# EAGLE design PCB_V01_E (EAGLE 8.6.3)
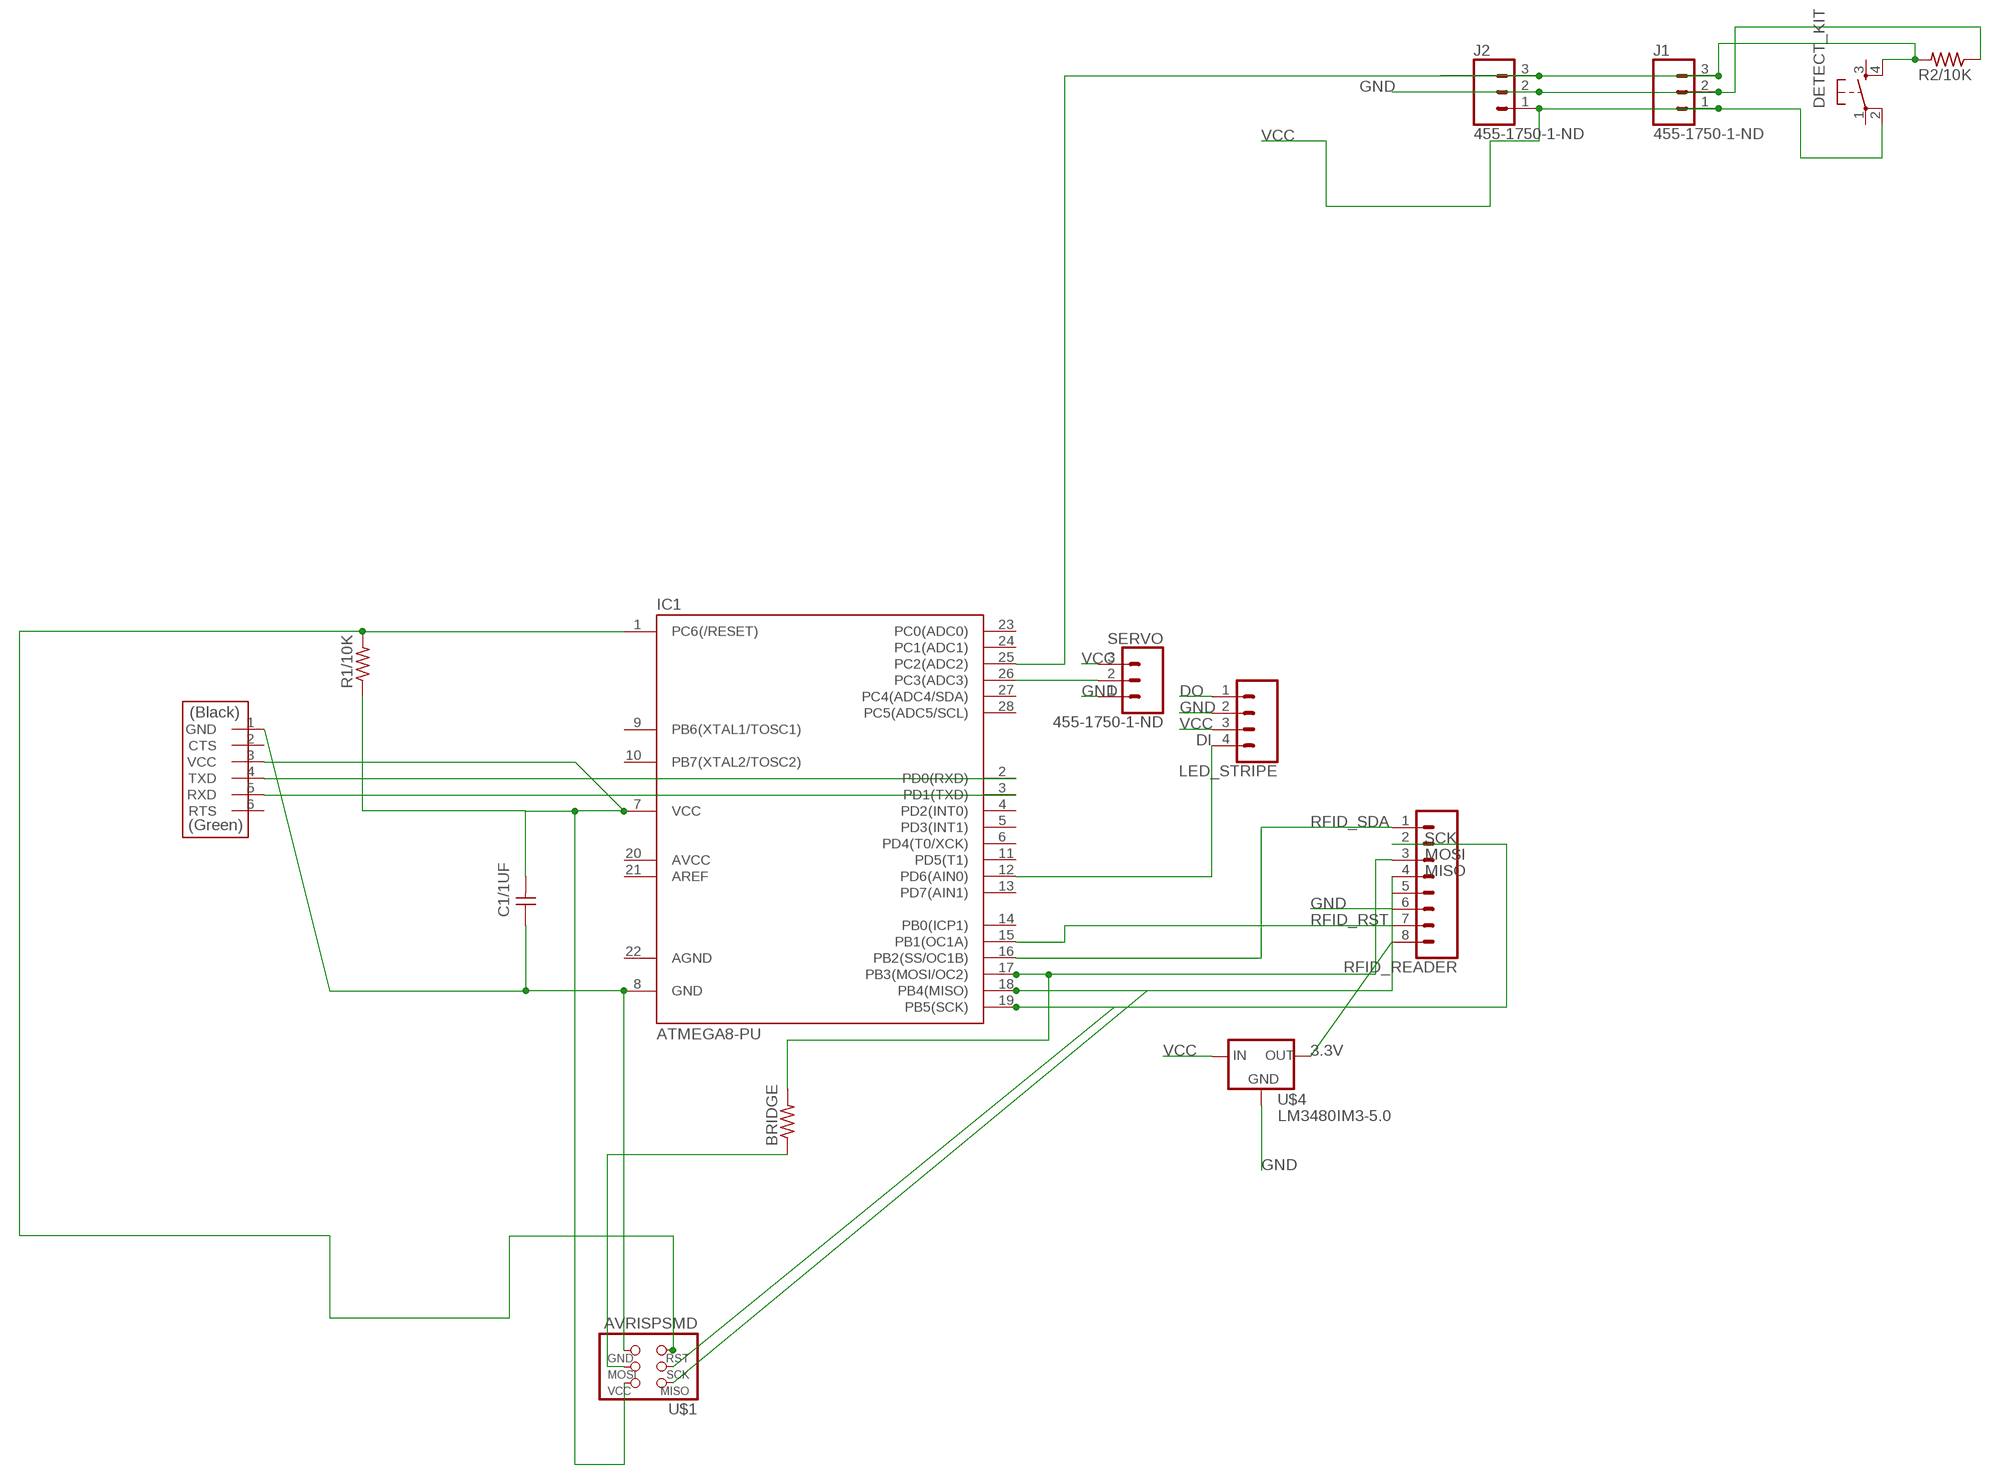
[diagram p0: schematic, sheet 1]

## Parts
BRIDGE  RES-US1206FAB  [R1206FAB]
C1/1UF  CAP-UNPOLARIZEDFAB  [C1206FAB]
DETECT_KIT  6MM_SWITCH6MM_SWITCH  [6MM_SWITCH]
IC1  ATMEGA8-PU  [DIL28-3]
J1  455-1750-1-ND  CONN_03  [1X03]
J2  455-1750-1-ND  CONN_03  [1X03]
LED_STRIPE  CONN_04  [1X04]
R1/10K  RES-US1206FAB  [R1206FAB]
R2/10K  RES-US1206FAB  [R1206FAB]
RFID_READER  CONN_08"  [1X08]
SERVO  455-1750-1-ND  CONN_03  [1X03]
U$1  AVRISPSMD  [2X03SMD]
U$2  FTDI-SMD-HEADER  [1X06SMD]
U$4  LM3480IM3-5.0  [SOT23]

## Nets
3.3V: RFID_READER.8 U$4.1(OUT)
DI: IC1.12(PD6(AIN0)) LED_STRIPE.4
DO: LED_STRIPE.1
GND: C1/1UF.1 IC1.8(GND) J1.2 J2.2 LED_STRIPE.2 R2/10K.1 RFID_READER.6 SERVO.1 U$1.6(GND) U$2.1(GND) U$4.3(GND)
MISO: IC1.18(PB4(MISO)) RFID_READER.4 U$1.1(MISO)
MOSI: BRIDGE.2 IC1.17(PB3(MOSI/OC2)) RFID_READER.3
N$1: BRIDGE.1 U$1.4(MOSI)
N$4: IC1.26(PC3(ADC3)) SERVO.2
N$8: IC1.3(PD1(TXD)) U$2.5(RXD)
N$9: IC1.2(PD0(RXD)) U$2.4(TXD)
N$10: DETECT_KIT.4(S1) IC1.25(PC2(ADC2)) J1.3 J2.3 R2/10K.2
N$14: IC1.1(PC6(/RESET)) R1/10K.2 U$1.5(RST)
RFID_RST: IC1.15(PB1(OC1A)) RFID_READER.7
RFID_SDA: IC1.16(PB2(SS/OC1B)) RFID_READER.1
SCK: IC1.19(PB5(SCK)) RFID_READER.2 U$1.3(SCK)
VCC: C1/1UF.2 DETECT_KIT.2(P1) IC1.7(VCC) J1.1 J2.1 LED_STRIPE.3 R1/10K.1 SERVO.3 U$1.2(VCC) U$2.3(VCC) U$4.2(IN)
Unconnected: DETECT_KIT.1(P) DETECT_KIT.3(S) IC1.4(PD2(INT0)) IC1.5(PD3(INT1)) IC1.6(PD4(T0/XCK)) IC1.9(PB6(XTAL1/TOSC1)) IC1.10(PB7(XTAL2/TOSC2)) IC1.11(PD5(T1)) IC1.13(PD7(AIN1)) IC1.14(PB0(ICP1)) IC1.20(AVCC) IC1.21(AREF) IC1.23(PC0(ADC0)) IC1.24(PC1(ADC1)) IC1.27(PC4(ADC4/SDA)) IC1.28(PC5(ADC5/SCL)) RFID_READER.5 U$2.2(CTS) U$2.6(RTS)

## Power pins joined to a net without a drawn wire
AGND: IC1.22(AGND)

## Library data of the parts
BRIDGE R1/10K R2/10K = fab:RES-US: Resistor (US Symbol)
C1/1UF = fab:CAP-UNPOLARIZED
DETECT_KIT = fab:6MM_SWITCH: OMRON SWITCH
IC1 = atmega8:ATMEGA8-PU
J1 J2 SERVO = SparkFun-Connectors:CONN_03: Multi connection point. Often used as Generic Header-pin footprint for 0.1 inch spaced/style header connections On any of the 0.1 inch spaced packages, you can populate with these: Break Away Headers - Straight (PRT-00116) Break Away Male Headers - Right Angle (PRT-00553) Female Headers (PRT-00115)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; PROD_ID: XXX-00000
LED_STRIPE = SparkFun-Connectors:CONN_04: Multi connection point. Often used as Generic Header-pin footprint for 0.1 inch spaced/style header connections On any of the 0.1 inch spaced packages, you can populate with these: Break Away Headers - Straight (PRT-00116) Break Away Male Headers - Right Angle (PRT-00553) Female Headers (PRT-00115)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; PROD_ID: CONN-09696
RFID_READER = SparkFun-Connectors:CONN_08: Multi connection point. Often used as Generic Header-pin footprint for 0.1 inch spaced/style header connections On any of the 0.1 inch spaced packages, you can populate with these: Break Away Headers - Straight (PRT-00116) Break Away Male Headers - Right Angle (PRT-00553) Female Headers (PRT-00115)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; PROD_ID: CONN-08438
U$1 = fab:AVRISP
U$2 = fab:FTDI-SMD-HEADER
U$4 = national_gaui:LM3480

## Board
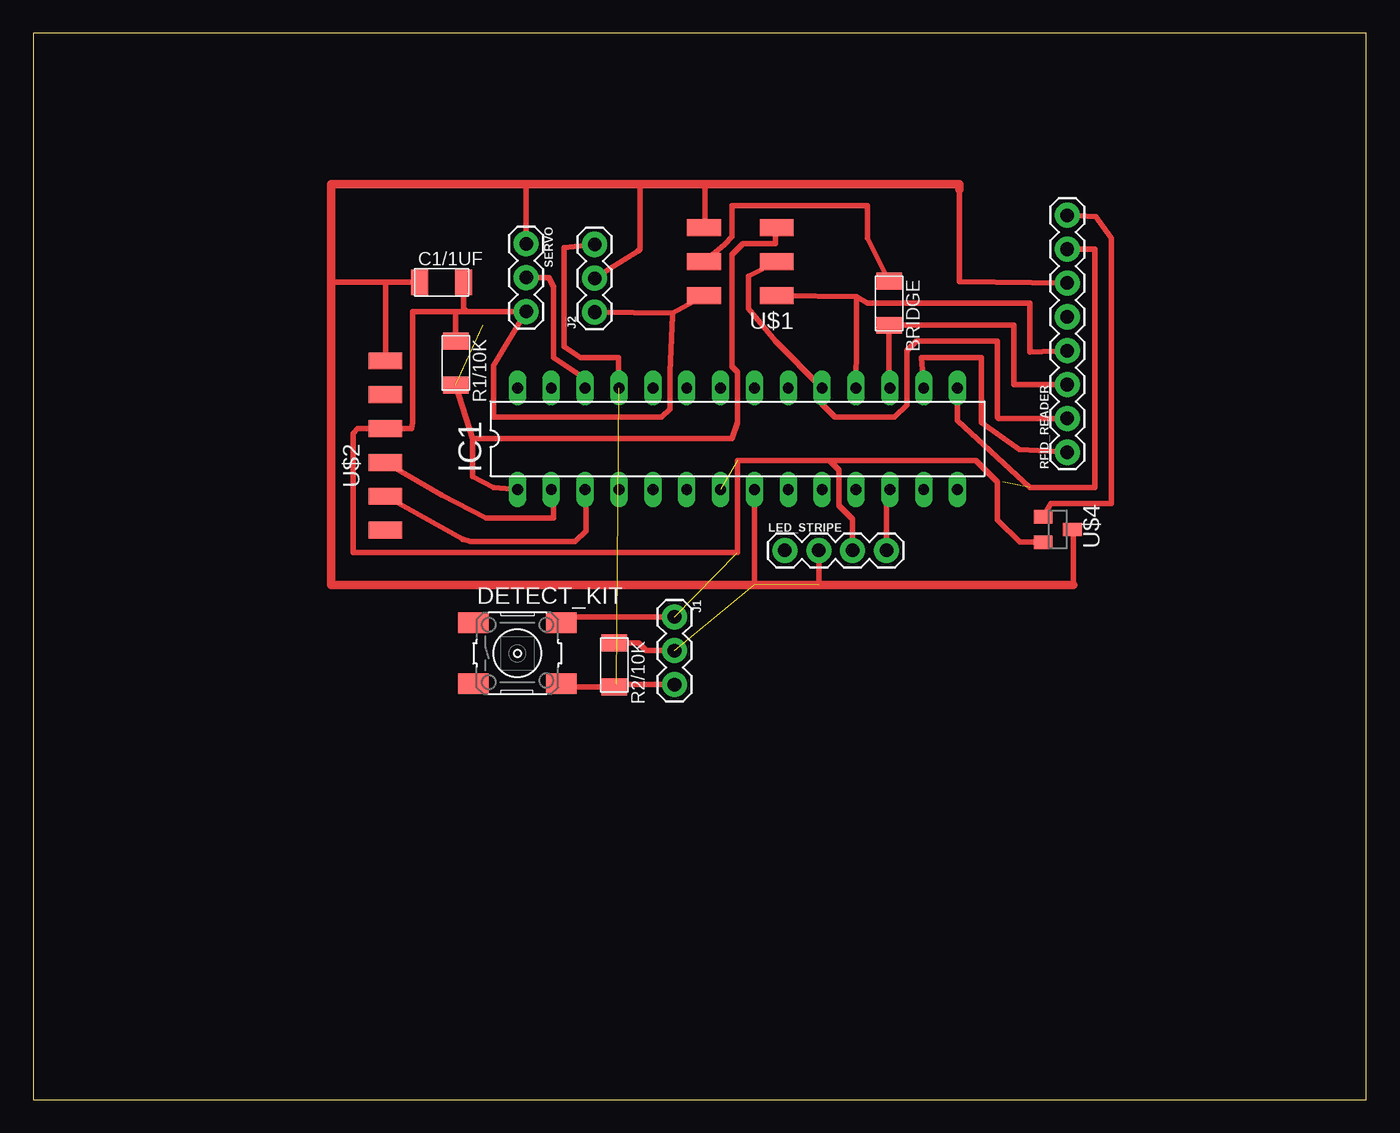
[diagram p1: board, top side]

Size 100 x 80 mm. Coordinates in mm from the lower left corner, seen from the top.
Outline: 0,0 100,0 100,80 0,80 0,0
Copper layers (1*16): Top 0.035mm / dielectric 1.5mm / Bottom 0.035mm
Design rules "default *": minimum track width 6mil, minimum drill 0.35mm, track to track 16mil, track to pad 16mil, pad to pad 16mil, via to via 16mil, smd to smd 16mil, copper to edge 40mil, drill to drill 6mil, minimum pad ring 10mil, minimum via ring 8mil, stop-mask expansion 4mil, vias tented up to drill 0mil, thermal gap 10mil

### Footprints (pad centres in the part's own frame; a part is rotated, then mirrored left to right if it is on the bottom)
R1206FAB = smd 1.27 x 1.905: 1 -1.651,0; 2 1.651,0
C1206FAB = smd 1.27 x 1.905: 1 -1.651,0; 2 1.651,0
6MM_SWITCH = smd 2.286 x 1.524: 1 -3.302,2.286; 2 3.302,2.286; 3 -3.302,-2.286; 4 3.302,-2.286
DIL28-3 = drill 0.813 long: 1 -16.51,-3.81; 2 -13.97,-3.81; 3 -11.43,-3.81; 4 -8.89,-3.81; 5 -6.35,-3.81; 6 -3.81,-3.81; 7 -1.27,-3.81; 8 1.27,-3.81; 9 3.81,-3.81; 10 6.35,-3.81; 11 8.89,-3.81; 12 11.43,-3.81; 13 13.97,-3.81; 14 16.51,-3.81; 15 16.51,3.81; 16 13.97,3.81; 17 11.43,3.81; 18 8.89,3.81; 19 6.35,3.81; 20 3.81,3.81; 21 1.27,3.81; 22 -1.27,3.81; 23 -3.81,3.81; 24 -6.35,3.81; 25 -8.89,3.81; 26 -11.43,3.81; 27 -13.97,3.81; 28 -16.51,3.81
1X03 = drill 1.016 pad 1.88: 1 0,0; 2 2.54,0; 3 5.08,0
1X04 = drill 1.016 pad 1.88: 1 0,0; 2 2.54,0; 3 5.08,0; 4 7.62,0
1X08 = drill 1.016 pad 1.88: 1 0,0; 2 2.54,0; 3 5.08,0; 4 7.62,0; 5 10.16,0; 6 12.7,0; 7 15.24,0; 8 17.78,0
2X03SMD = smd 2.54 x 1.27: 1 -2.54,2.54; 2 2.92,2.54; 3 -2.54,0; 4 2.92,0; 5 -2.54,-2.54; 6 2.92,-2.54
1X06SMD = smd 2.54 x 1.27: 1 0,6.35; 2 0,3.81; 3 0,1.27; 4 0,-1.27; 5 0,-3.81; 6 0,-6.35
SOT23 = smd 1 x 1.4: 1 -0.95,-1.1; 2 0.95,-1.1; 3 0,1.1

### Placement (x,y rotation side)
BRIDGE  64.21,59.74 270 top
C1/1UF  30.63,61.32 0 top
DETECT_KIT  36.32,33.48 0 top
IC1  52.83,49.58 0 top
J1  48.11,36.22 270 top
J2  42.11,59.08 90 top
LED_STRIPE  56.39,41.2 0 top
R1/10K  31.7,55.27 270 top
R2/10K  43.59,32.61 270 top
RFID_READER  77.57,48.56 90 top
SERVO  36.98,64.21 270 top
U$1  53.24,62.86 180 top
U$2  26.42,49.07 0 top
U$4  76.86,42.77 270 top

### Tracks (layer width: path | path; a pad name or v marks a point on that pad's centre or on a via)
3.3V
  Top 0.406: 75.95,43.91 U$4.1 76.33,44.7 80.87,44.7 80.87,64.62 79.7,66.24 RFID_READER.8
DI
  Top 0.406: LED_STRIPE.4 64.01,45.52 IC1.12
GND  (2 unrouted)
  Top 0.406: U$1.6 50.39,65.48 50.39,68.68 | SERVO.1 36.98,68.68 | J2.2 45.36,63.65 45.52,63.8 45.52,68.68 | RFID_READER.6 69.49,61.37 69.49,68.68 | 54.1,45.21 IC1.8 54.1,38.66 54.05,38.61 | LED_STRIPE.2 58.93,38.61 | J1.2 45.97,33.68 45.39,34.27 R2/10K.1 | U$4.3 78.03,42.77 78.03,38.61 | 22.35,61.37 22.35,61.32 26.42,61.32 | 26.42,61.32 C1/1UF.1 | U$2.1 26.42,61.32
  Top 0.635: 69.49,68.28 69.49,68.68 50.39,68.68 45.52,68.68 36.98,68.68 22.35,68.68 22.35,61.37 22.35,38.61 58.93,38.61 78.03,38.61
MISO
  Top 0.406: U$1.1 61.77,60.25 | 61.77,60.25 61.75,56.9 IC1.18 | RFID_READER.4 74.78,56.08 74.78,59.74 62.59,59.74 61.77,60.25
MOSI
  Top 0.406: IC1.17 64.35,53.39 64.21,53.52 BRIDGE.2 66.62,58.09 73.56,58.12 73.56,53.65 RFID_READER.3
N$1
  Top 0.406: U$1.4 51.84,64.16 52.43,64.74 52.43,67.06 62.59,67.06 62.59,64.64 BRIDGE.1
N$4
  Top 0.406: SERVO.2 38.71,61.67 39.01,60.96 39.01,55.68 41.4,54.1 IC1.26
N$8
  Top 0.406: U$2.5 32.21,42.04 | 32.21,42.04 32.26,42.01 | 32.21,42.04 32.79,41.86 40.64,41.86 41.45,42.67 41.45,45.72 IC1.3
N$9
  Top 0.406: U$2.4 30.63,45.36 33.98,43.64 39.01,43.64 39.01,45.62 IC1.2
N$10  (1 unrouted)
  Top 0.406: J2.3 39.83,63.91 39.83,56.49 41.05,55.68 43.89,55.68 43.94,53.59 IC1.25 | J1.3 43.76,31.14 R2/10K.2 39.85,30.96 DETECT_KIT.4
N$14  (1 unrouted)
  Top 0.406: R1/10K.2 32.94,49.58 | 32.94,49.58 32.94,46.76 34.54,45.92 IC1.1 | U$1.5 55.68,65.3 55.68,64.21 53.24,64.21 52.43,63.4 52.43,54.98 52.83,54.58 52.83,50.8 52.43,49.58 32.94,49.58
RFID_RST  (1 unrouted)
  Top 0.406: RFID_READER.7 79.65,63.8 79.65,45.92 74.78,45.92 69.34,50.95 IC1.15
RFID_SDA
  Top 0.406: RFID_READER.1 73.97,48.77 71.12,50.8 71.12,55.68 66.65,55.68 IC1.16
SCK
  Top 0.406: U$1.3 53.65,61.77 53.65,59.33 55.68,56.9 IC1.19 59.18,52.17 60.15,51.21 64.62,51.21 65.53,52.12 65.53,56.19 66.24,56.9 72.34,56.9 72.34,51.21 72.44,51.1 RFID_READER.2
VCC  (2 unrouted)
  Top 0.406: 29.67,59.13 28.45,59.13 28.45,50.8 28.4,50.34 U$2.3 24.33,50.34 23.98,49.99 23.98,41.05 52.83,41.05 52.83,47.95 59.74,47.95 | 29.67,59.13 31.7,59.13 | 31.7,59.13 SERVO.3 34.54,55.07 34.54,51.21 47.14,51.21 47.75,51.82 47.75,54.58 47.97,58.83 47.97,59.01 | J2.1 47.97,59.01 | 47.97,59.01 50.29,60.3 U$1.2 | LED_STRIPE.3 61.47,43.57 60.45,44.58 60.45,47.24 59.74,47.95 | 29.67,59.13 29.64,59.11 | 59.74,47.95 70.71,47.95 72.34,46.33 72.34,43.48 74,41.82 U$4.2 | R1/10K.1 31.7,59.13 | C1/1UF.2 32.28,59.36 32.51,59.13 | J1.1 40.08,36.22 DETECT_KIT.2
